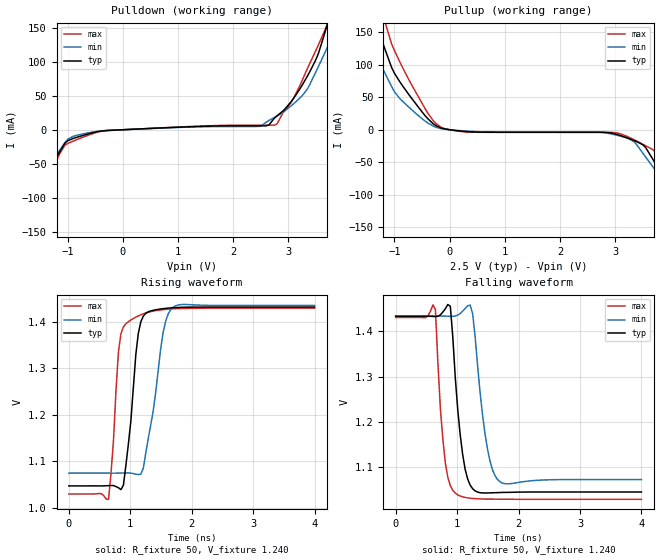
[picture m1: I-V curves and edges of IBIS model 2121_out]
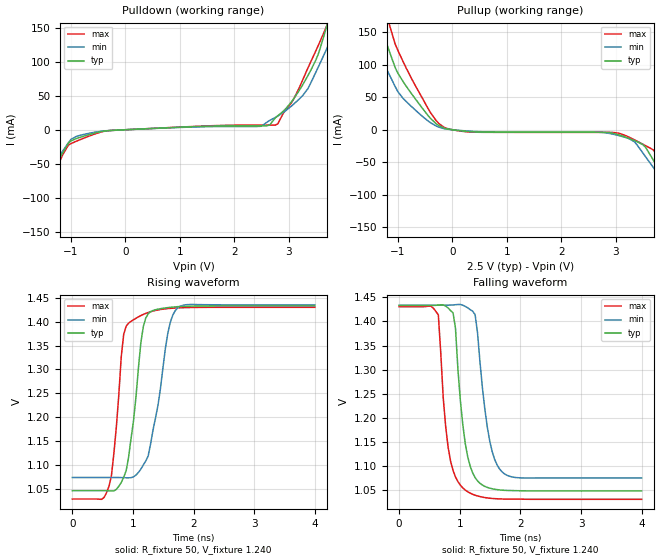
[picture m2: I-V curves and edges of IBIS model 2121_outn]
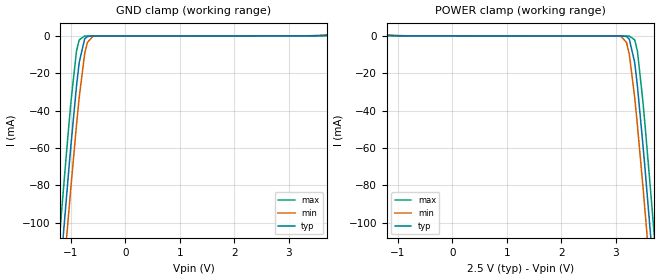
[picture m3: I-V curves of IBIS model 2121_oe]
| IBIS File eg2121l2.ibs
[IBIS ver]   3.2
[File name]   eg2121l2.ibs
[File Rev]   5
[Date]   June 23,2011
[Source]   Circiuts Simulation for EG-2121CA LVDS by HSPICE
|   Component EG-2121CA LVDS
[Component]   EG-2121L
|   (175M<f<250M, 350M<f<500M)
[Manufacturer]   Epson Toyocom Corp.
[Package]
| variable   typ   min   max
R_pkg   1.04   NA   NA
L_pkg   1.98nH  NA   NA
C_pkg   3.71pF  NA   NA
[Pin]   signal_name   model_name   R_pin   L_pin   C_pin
1   oe   2121_oe   NA   NA   NA
4   out   2121_out   1.04   1.98n   3.71p
5   outn   2121_outn   1.04   1.98n   3.71p
6   vdd   POWER   NA   NA   NA
3   vss   GND   NA   NA   NA
[Diff Pin] inv_pin vdiff   tdelay_typ
4   5   0   0
| Models and submodels in the file (3): 2121_out (Output), 2121_outn (Output), 2121_oe (Input)
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[Model]   2121_out
Model_type Output
Enable Active-High
Polarity Non-Inverting
Vref=1.240
Vmeas=1.240
Rref=50
Cref=0
C_comp   3.77p   3.77p   3.77p
[Temperature Range] 25   85   -40
[Voltage Range]   2.5   2.35   2.65
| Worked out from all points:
|   slope of the pulldown table from 0 to 0.375 V, typ, clamps not added: 260 ohm
|   slope of the pullup table from 0 to 0.375 V, typ, clamps not added: 120 ohm
|   falling waveform, R_fixture 50, V_fixture 1.240: 20-80 % time 152ps typ, 179ps min, 128ps max; typ from 1.43 V to 1.05 V
|   rising waveform, R_fixture 50, V_fixture 1.240: 20-80 % time 155ps typ, 229ps min, 115ps max; typ from 1.05 V to 1.43 V
[Pullup]
-2.5V     463.7mA    342.9mA    607.2mA
-1.6V     229.3mA    162.4mA    307.7mA
-1.3V     155mA      109.2mA    208.3mA
-1.15V    118.9mA    83.37mA    159.7mA
-900mV    73.47mA    47.8mA     103.9mA
-250mV    6.37mA     3.952mA    9.708mA
2.75V     -3.907mA   -4.077mA   -4.035mA
3.35V     -16.93mA   -18.79mA   -15.7mA
3.7V      -47.82mA   -58.94mA   -31.6mA
4.45V     -147.9mA   -142.4mA   -153.5mA
4.6V      -169.3mA   -159.4mA   -181.7mA
5V        -223.4mA   -202.7mA   -254.3mA
[Pulldown]
-2.5V     -242.9mA   -203.9mA   -301.8mA
-2.05V    -176.9mA   -149.4mA   -216.9mA
-1.9V     -153.3mA   -130.1mA   -186.5mA
-1.75V    -129mA     -110.3mA   -155.4mA
-1.15V    -33.42mA   -30.96mA   -36.45mA
-900mV    -12.88mA   -9.74mA    -16.81mA
-300mV    -1.239mA   -1.161mA   -1.287mA
2.75V     17.22mA    18mA       6.76mA
3.35V     79.42mA    60.21mA    90.67mA
3.7V      152.8mA    119.7mA    153.6mA
3.95V     219.9mA    164.3mA    229.4mA
5V        520.5mA    381.8mA    575.7mA
[Falling Waveform]
R_fixture=50
V_fixture=1.240
V_fixture_min=1.254
V_fixture_max=1.230
0s        1.433V     1.434V     1.431V
646.5ps   1.433V     1.434V     1.449V
808.1ps   1.45V      1.434V     1.11V
888.9ps   1.455V     1.433V     1.06V
969.7ps   1.298V     1.434V     1.044V
1.172ns   1.074V     1.457V     1.033V
1.253ns   1.053V     1.439V     1.032V
1.495ns   1.044V     1.14V      1.03V
1.697ns   1.045V     1.068V     1.03V
4ns       1.046V     1.073V     1.03V
[Rising Waveform]
R_fixture=50
V_fixture=1.240
V_fixture_min=1.254
V_fixture_max=1.230
0s        1.047V     1.074V     1.029V
646.5ps   1.047V     1.074V     1.018V
808.1ps   1.043V     1.074V     1.336V
888.9ps   1.048V     1.075V     1.389V
969.7ps   1.137V     1.075V     1.401V
1.091ns   1.33V      1.072V     1.41V
1.172ns   1.4V       1.072V     1.415V
1.535ns   1.429V     1.377V     1.427V
1.697ns   1.431V     1.432V     1.428V
4ns       1.432V     1.436V     1.43V
[Ramp]
R_load=50
dV/dt_r   2.312E-1/1.525E-10   NA   NA
dV/dt_f   2.324E-1/1.518E-10   NA   NA
|[End   2121_out
[Model]   2121_outn
Model_type Output
Enable Active-High
Polarity Inverting
Vref=1.240
Vmeas=1.240
Rref=50
Cref=0
C_comp   3.77p   3.77p   3.77p
[Temperature Range] 25   85   -40
[Voltage Range]   2.5   2.35   2.65
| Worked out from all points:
|   slope of the pulldown table from 0 to 0.375 V, typ, clamps not added: 260 ohm
|   slope of the pullup table from 0 to 0.375 V, typ, clamps not added: 120 ohm
|   falling waveform, R_fixture 50, V_fixture 1.240: 20-80 % time 179ps typ, 200ps min, 169ps max; typ from 1.43 V to 1.05 V
|   rising waveform, R_fixture 50, V_fixture 1.240: 20-80 % time 194ps typ, 265ps min, 155ps max; typ from 1.05 V to 1.43 V
[Pullup]
-2.5V     463.7mA    342.9mA    607.2mA
-1.6V     229.3mA    162.4mA    307.7mA
-1.3V     155mA      109.2mA    208.3mA
-1.15V    118.9mA    83.37mA    159.7mA
-900mV    73.47mA    47.8mA     103.9mA
-250mV    6.37mA     3.952mA    9.708mA
2.75V     -3.907mA   -4.077mA   -4.035mA
3.35V     -16.93mA   -18.79mA   -15.7mA
3.7V      -47.82mA   -58.94mA   -31.6mA
4.45V     -147.9mA   -142.4mA   -153.5mA
4.6V      -169.3mA   -159.4mA   -181.7mA
5V        -223.4mA   -202.7mA   -254.3mA
[Pulldown]
-2.5V     -242.9mA   -203.9mA   -301.8mA
-2.05V    -176.9mA   -149.4mA   -216.9mA
-1.9V     -153.3mA   -130.1mA   -186.5mA
-1.75V    -129mA     -110.3mA   -155.4mA
-1.15V    -33.42mA   -30.96mA   -36.45mA
-900mV    -12.88mA   -9.74mA    -16.81mA
-300mV    -1.239mA   -1.161mA   -1.287mA
2.75V     17.22mA    18mA       6.76mA
3.35V     79.42mA    60.21mA    90.67mA
3.7V      152.8mA    119.7mA    153.6mA
3.95V     219.9mA    164.3mA    229.4mA
5V        520.5mA    381.8mA    575.7mA
[Falling Waveform]
R_fixture=50
V_fixture=1.240
V_fixture_min=1.254
V_fixture_max=1.230
0s        1.433V     1.434V     1.431V
646.5ps   1.434V     1.434V     1.414V
767.7ps   1.432V     1.434V     1.181V
888.9ps   1.418V     1.434V     1.09V
929.3ps   1.386V     1.435V     1.077V
1.091ns   1.146V     1.431V     1.049V
1.253ns   1.075V     1.414V     1.039V
1.455ns   1.055V     1.18V      1.033V
1.697ns   1.049V     1.087V     1.031V
4ns       1.047V     1.075V     1.03V
[Rising Waveform]
R_fixture=50
V_fixture=1.240
V_fixture_min=1.254
V_fixture_max=1.230
0s        1.047V     1.074V     1.029V
606.1ps   1.046V     1.074V     1.056V
686.9ps   1.046V     1.074V     1.125V
848.5ps   1.075V     1.074V     1.373V
929.3ps   1.117V     1.073V     1.397V
1.131ns   1.356V     1.092V     1.413V
1.293ns   1.421V     1.145V     1.421V
1.576ns   1.429V     1.376V     1.427V
1.737ns   1.431V     1.428V     1.429V
4ns       1.433V     1.435V     1.43V
[Ramp]
R_load=50
dV/dt_r   2.318E-1/1.944E-10   NA   NA
dV/dt_f   2.316E-1/1.772E-10   NA   NA
|[End   2121_outn
[Model]   2121_oe
Model_type Input
Vinh=1.75
Vinl=0.75
C_comp   3p   3p   3p
[Temperature Range] 25   85   -40
[Voltage Range]   2.5   2.35   2.65
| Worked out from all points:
|   GND clamp passes 1 mA (typ) near -0.73 V on its own axis
|   POWER clamp passes 1 mA (typ) near -1.64 V on its own axis
[GND Clamp]
-2.5V     -614.1mA   -635.2mA   -592.4mA
-1.2V     -127.3mA   -150mA     -103.5mA
-1.15V    -109.5mA   -132.2mA   -85.68mA
-1.05V    -74.64mA   -97.23mA   -51.09mA
-1V       -57.87mA   -80.21mA   -34.8mA
-900mV    -26.94mA   -47.79mA   -8.114mA
-850mV    -14.21mA   -32.96mA   -2.138mA
-750mV    -1.674mA   -9.601mA   -76.22uA
-700mV    -312uA     -3.576mA   -59.18uA
-550mV    -37.86uA   -75.63uA   -57.57uA
3.35V     44.48uA    81.69uA    49.55uA
5V        2.629mA    2.956mA    2.308mA
[POWER Clamp]
-2.5V     2.629mA    2.956mA    2.308mA
-850mV    44.48uA    81.69uA    49.55uA
3.05V     -37.86uA   -75.63uA   -57.57uA
3.2V      -312uA     -3.576mA   -59.18uA
3.25V     -1.674mA   -9.601mA   -76.22uA
3.35V     -14.21mA   -32.96mA   -2.138mA
3.4V      -26.94mA   -47.79mA   -8.114mA
3.5V      -57.87mA   -80.21mA   -34.8mA
3.55V     -74.64mA   -97.23mA   -51.09mA
3.65V     -109.5mA   -132.2mA   -85.68mA
3.7V      -127.3mA   -150mA     -103.5mA
5V        -614.1mA   -635.2mA   -592.4mA
